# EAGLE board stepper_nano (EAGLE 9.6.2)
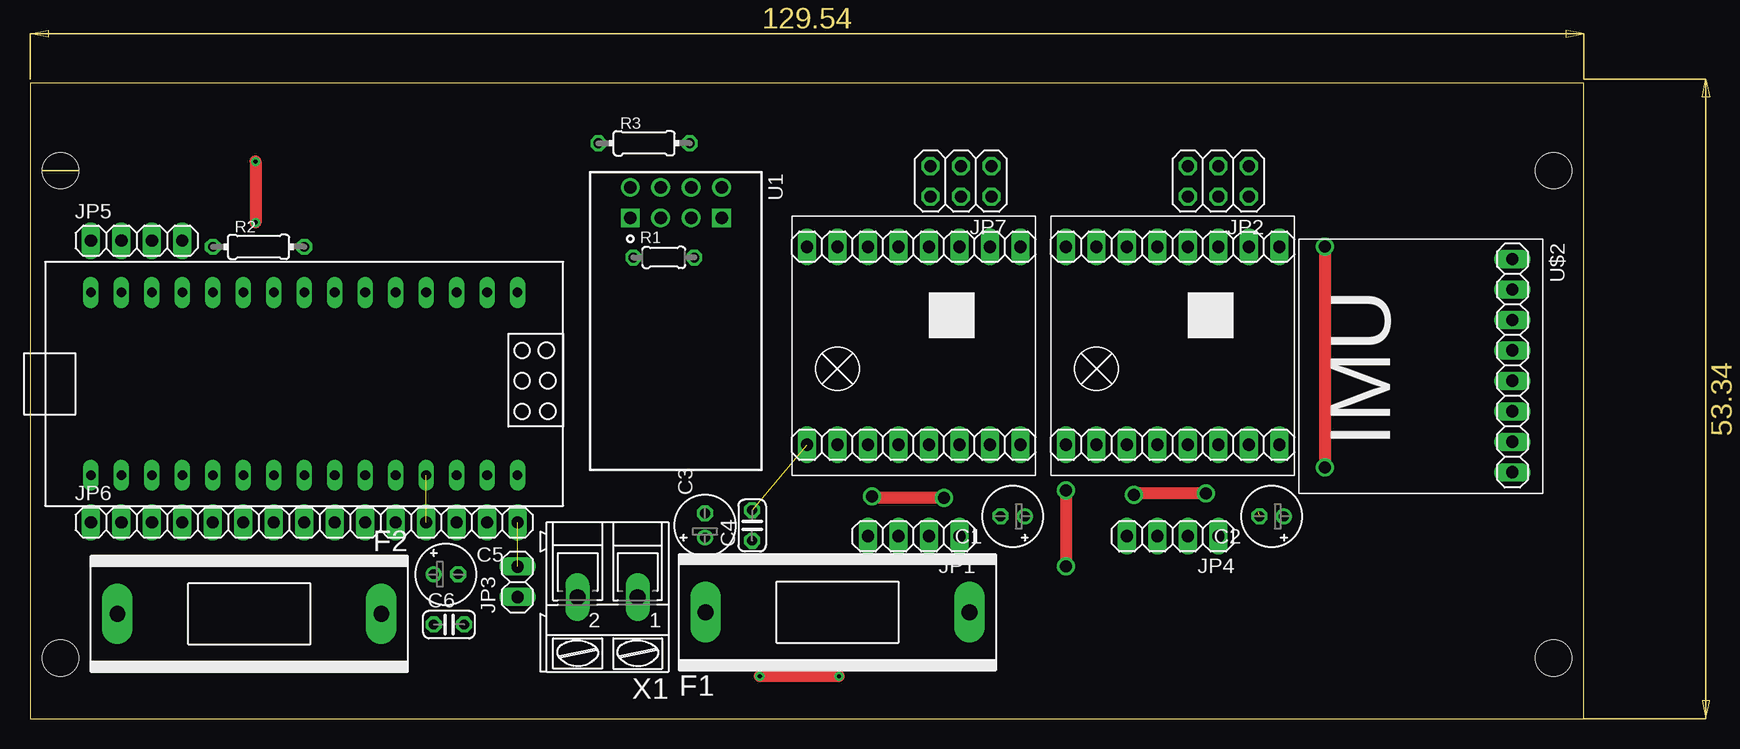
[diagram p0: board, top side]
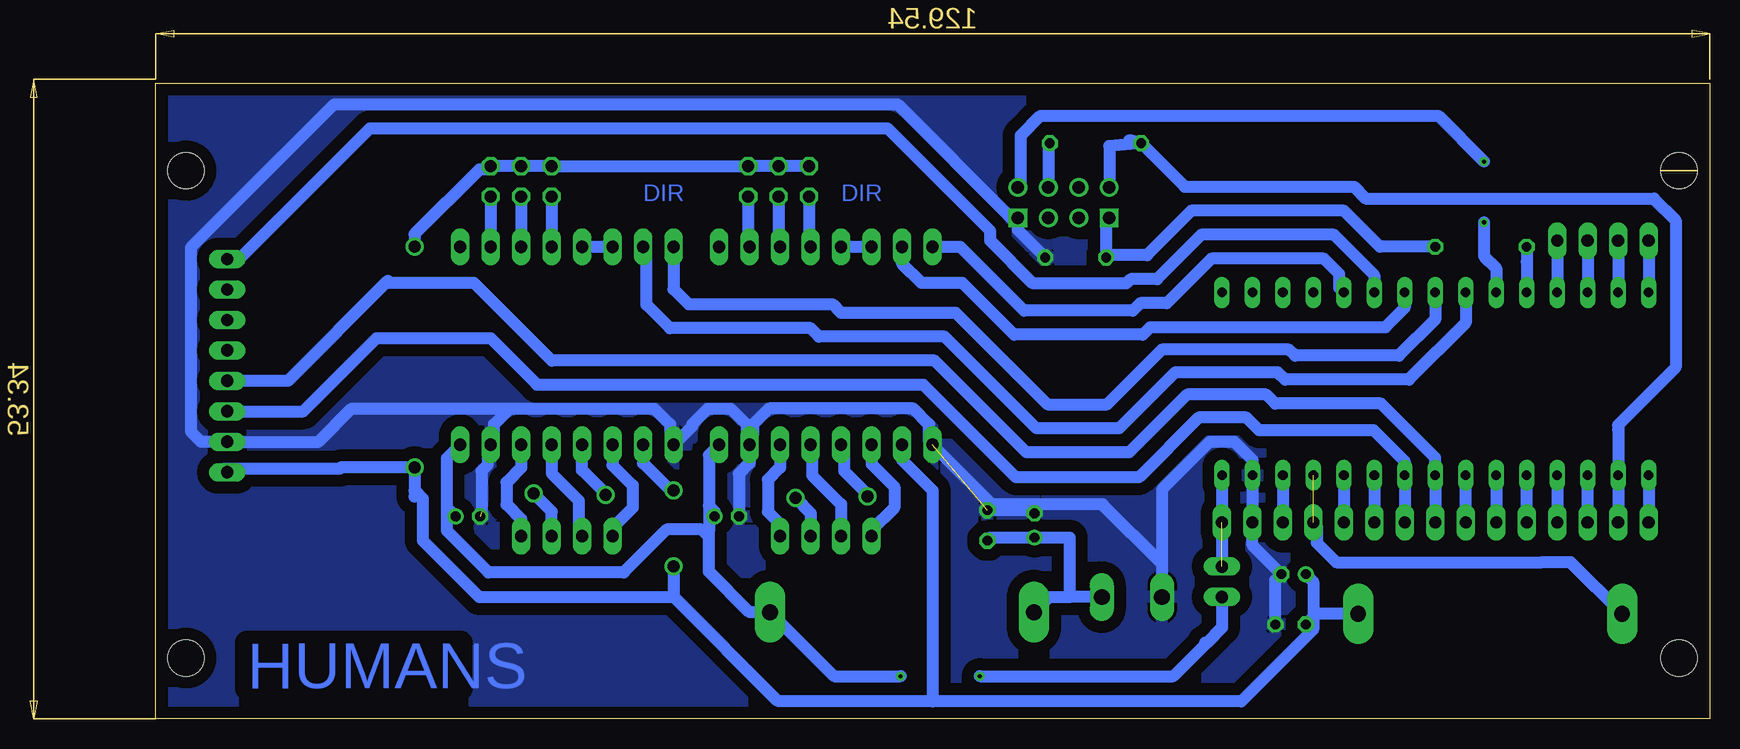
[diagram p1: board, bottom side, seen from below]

Size 140 x 57.45 mm. Coordinates in mm from the lower left corner, seen from the top.
Outline: 0,0 129.52,0 129.52,53.01 0,53.01 0,0
Copper layers (1*16): Top 0.035mm / dielectric 1.5mm / Bottom 0.035mm
Design rules "default *": minimum track width 6mil, minimum drill 0.35mm, track to track 1mm, track to pad 1mm, pad to pad 1mm, via to via 6mil, smd to smd 6mil, copper to edge 40mil, drill to drill 6mil, minimum pad ring 10mil, minimum via ring 8mil, stop-mask expansion 4mil, vias tented up to drill 0mil, thermal gap 10mil
Holes 3 mm at 2.54,45.72 2.54,5.08 127,5.08 127,45.72

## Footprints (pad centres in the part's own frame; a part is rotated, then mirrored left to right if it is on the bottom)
E2-5 = drill 0.813 pad 1.27: + -1.016,0 | drill 0.813 pad 1.27 octagon: - 1.016,0
C025-024X044 = drill 0.813 octagon: 1 -1.27,0; 2 1.27,0
SH22 = drill 1.321 pad 2.54 long: 1 -10.998,0; 2 10.998,0
1X04 = drill 1.016 long: 1 -3.81,0; 2 -1.27,0; 3 1.27,0; 4 3.81,0
2X03 = drill 1.016 octagon: 1 -2.54,-1.27; 2 -2.54,1.27; 3 0,-1.27; 4 0,1.27; 5 2.54,-1.27; 6 2.54,1.27
1X02 = drill 1.016 long: 1 -1.27,0; 2 1.27,0
1X15 = drill 1.016 long: 1 -17.78,0; 2 -15.24,0; 3 -12.7,0; 4 -10.16,0; 5 -7.62,0; 6 -5.08,0; 7 -2.54,0; 8 0,0; 9 2.54,0; 10 5.08,0; 11 7.62,0; 12 10.16,0; 13 12.7,0; 14 15.24,0; 15 17.78,0
0204/5 = drill 0.813 octagon: 1 -2.54,0; 2 2.54,0
0204/7 = drill 0.813 octagon: 1 -3.81,0; 2 3.81,0
XCVR_ESP8266-01/ESP-01 = drill 1.05 square: 1 0,-3.81; 4 0,3.81 | drill 1.05: 2 0,-1.27; 3 0,1.27; 5 -2.54,3.81; 6 -2.54,1.27; 7 -2.54,-1.27; 8 -2.54,-3.81
NANO = drill 0.8 long: 3.3V -10.16,24.13; 5V -10.16,-1.27; A0 -10.16,19.05; A1 -10.16,16.51; A2 -10.16,13.97; A3 -10.16,11.43; A4 -10.16,8.89; A5 -10.16,6.35; A6 -10.16,3.81; A7 -10.16,1.27; AREF -10.16,21.59; D2 5.08,1.27; D3 5.08,3.81; D4 5.08,6.35; D5 5.08,8.89; D6 5.08,11.43; D7 5.08,13.97; D8 5.08,16.51; D9 5.08,19.05; D10 5.08,21.59; D11 5.08,24.13; D12 5.08,26.67; D13 -10.16,26.67; GND -10.16,-6.35; GND1 5.08,-1.27; RAW -10.16,-8.89; RST -10.16,-3.81; RST1 5.08,-3.81; RX1 5.08,-6.35; TX0 5.08,-8.89
IMU_GY521 = drill 1.016 long: ADO -6.35,0; GND 6.35,0; INT -8.89,0; SCL 3.81,0; SDA 1.27,0; VCC 8.89,0; XCL -3.81,0; XDA -1.27,0
A4988-DRIVER = drill 1.016 long: 1 -7.62,8.89; 2 -7.62,6.35; 3 -7.62,3.81; 4 -7.62,1.27; 5 -7.62,-1.27; 6 -7.62,-3.81; 7 -7.62,-6.35; 8 -7.62,-8.89; 9 8.89,8.89; 10 8.89,6.35; 11 8.89,3.81; 12 8.89,1.27; 13 8.89,-1.27; 14 8.89,-3.81; 15 8.89,-6.35; 16 8.89,-8.89
AK300/2 = drill 1.321 long: 1 -2.515,0; 2 2.489,0

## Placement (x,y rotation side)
C1  [E2-5]  81.92,16.89 180 top
C2  [E2-5]  103.5,16.89 180 top
C3  [E2-5]  56.26,16.13 90 top
C4  [C025-024X044]  60.2,16.13 90 top
C5  [E2-5]  34.67,12.07 0 top
C6  [C025-024X044]  34.92,7.87 0 top
F1  1A  [SH22]  67.31,8.89 0 top
F2  300mA  [SH22]  18.29,8.76 180 top
JP1  [1X04]  73.66,15.24 180 top
JP2  [2X03]  99.06,44.83 180 top
JP3  [1X02]  40.64,11.43 90 top
JP4  [1X04]  95.25,15.24 180 top
JP5  [1X04]  8.89,39.88 0 top
JP6  [1X15]  22.86,16.38 0 top
JP7  [2X03]  77.6,44.83 180 top
R1  [0204/5]  52.83,38.48 0 top
R2  [0204/7]  19.05,39.37 0 top
R3  [0204/7]  51.18,48.01 0 top
U1  ESP8266-01/ESP-01  [XCVR_ESP8266-01/ESP-01]  53.85,41.78 270 top
U$1  ARDUINO_NANO  [NANO]  31.75,30.48 90 top
U$2  IMU-MPU  [IMU_GY521]  123.57,29.46 270 top
U$3  [A4988-DRIVER]  73.66,31.75 270 top
U$4  [A4988-DRIVER]  95.25,31.75 270 top
X1  [AK300/2]  48.13,10.16 180 top

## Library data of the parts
C1-C6 = rcl; SPICEPREFIX: C
F1 F2 = fuse; OC_FARNELL: unknown; OC_NEWARK: unknown
JP1-JP7 = pinhead
R1-R3 = rcl; SPICEPREFIX: R
U1 = mohamed-eagle; AVAILABILITY: Not in stock; DESCRIPTION: MakerFocus 4pcs ESP8266 ESP-01 Serial Wireless WiFi Transceiver Receiver Module 1MB SPI Flash DC3.0-3.6V Internet of Things WiFi Module Board Compatible with Ar duino; MF: AI-Thinker; MP: ESP8266-01/ESP-01; PACKAGE: Non-Standard AI-Thinker; PRICE: None
U$1-U$4 = mohamed-eagle
X1 = con-ptr500; OC_FARNELL: unknown; OC_NEWARK: unknown

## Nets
3.3V: JP6.2 R3.1 U1.8 U$1.3.3V
5V: C5.+ C6.1 F2.1 JP2.1 JP2.3 JP2.5 JP7.1 JP7.3 JP7.5 U$2.VCC U$3.15 U$4.15
BAT+12: C1.+ C2.+ F1.2 JP3.1 U$3.9 U$4.9
D7: U1.5 U$1.D7
D8: R2.1 U$1.D8
DIR: U$1.D2 U$3.8
DIR1: U$1.D5 U$4.8
FUSE-5V: F2.2 JP6.12 U$1.5V
GND: C1.- C2.- C3.- C4.2 C5.- C6.2 JP6.14 R1.2 U1.4 U$1.GND U$2.GND U$3.10 U$3.16 U$4.10 U$4.16 X1.2
IMU-INT: U$1.D3 U$2.INT
N$1: JP1.1 U$3.11
N$2: JP1.4 U$3.14
N$3: JP1.2 U$3.13
N$4: JP1.3 U$3.12
N$5: JP4.1 U$4.11
N$6: JP4.4 U$4.14
N$7: JP4.2 U$4.13
N$8: JP4.3 U$4.12
N$9: JP7.2 U$3.2
N$10: JP7.4 U$3.3
N$11: JP7.6 U$3.4
N$12: U$3.5 U$3.6
N$13: JP2.2 U$4.2
N$14: JP2.4 U$4.3
N$15: JP2.6 U$4.4
N$16: U$4.5 U$4.6
N$17: R3.2 U1.6
N$18: JP3.2 JP6.15 U$1.RAW
N$19: JP5.4 U$1.D9
N$20: JP5.3 U$1.D10
N$21: R1.1 R2.2 U1.1
N$22: JP5.2 U$1.D11
N$23: JP5.1 U$1.D12
N$24: JP6.1 U$1.D13
N$25: JP6.3 U$1.AREF
N$26: JP6.4 U$1.A0
N$27: JP6.5 U$1.A1
N$28: JP6.6 U$1.A2
N$29: JP6.7 U$1.A3
N$30: JP6.10 U$1.A6
N$31: JP6.11 U$1.A7
N$32: JP6.13 U$1.RST
N$34: C3.+ C4.1 F1.1 X1.1
SCL: JP6.9 U$1.A5 U$2.SCL
SDA: JP6.8 U$1.A4 U$2.SDA
STEP: U$1.D4 U$3.7
STEP1: U$1.D6 U$4.7

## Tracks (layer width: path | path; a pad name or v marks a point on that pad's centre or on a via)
3.3V
  Bottom 1: R3.1 50.04,47.76 U1.8 | R3.1 48.39,48.26 | 7.62,24.13 U$1.3.3V | U$1.3.3V JP6.2 | R3.1 43.73,44.37 29.64,44.37 28.68,43.4 4.64,43.4 2.82,41.58 2.82,29.31 7.62,24.51 U$1.3.3V
5V  (via drill 1)
  Top 1: v86.36,19.05 v86.36,12.7 | v107.95,39.37 v107.95,20.99
  Bottom 1: 33.02,7.62 33.02,11.43 C5.+ | 33.02,7.62 33.02,7.46 39.04,1.45 64.77,1.45 64.77,1.52 | JP7.5 JP7.3 JP7.1 JP2.5 JP2.3 JP2.1 101.88,45.82 102.54,45.82 107.95,40.41 v107.95,39.37 | U$4.15 88.9,21.34 86.61,19.05 v86.36,19.05 | v86.36,12.7 86.36,10.16 | U$2.VCC 123.85,20.85 114.16,20.85 114.02,20.99 v107.95,20.99 107.95,19.05 | 107.95,19.05 107.95,18.54 | 33.02,7.62 33.4,7.62 C6.1 32.77,8.76 F2.1 | U$3.15 67.31,21.59 64.77,19.05 64.77,1.52 | 107.95,19.05 107.26,18.36 107.26,14.87 102.55,10.16 86.36,10.16 | 86.36,10.16 77.72,1.52 64.77,1.52
BAT+12  (via drill 0.35)
  Top 1: v67.44,3.56 v60.83,3.56
  Bottom 1: 41.91,6.35 42.04,6.35 | 103.86,23.14 U$4.9 105.26,21.74 105.26,17.63 | U$3.9 83.42,22 83.42,17.78 | 105.26,17.63 105.26,15.7 101.78,12.22 90.5,12.22 86.92,15.8 84.02,15.8 83.64,15.42 83.42,15.65 | C2.+ 105.26,17.63 | 83.42,17.78 83.42,15.65 | C1.+ 82.93,17.3 83.42,17.78 | 83.42,15.65 83.42,12.3 80.01,8.89 F1.2 72.97,3.56 v67.44,3.56 | v60.83,3.56 44.7,3.56 41.91,6.35 | JP3.1 40.64,7.62 41.91,6.35
D7  (via drill 0.35)
  Top 1: v18.8,46.48 v18.8,41.4
  Bottom 1: U$1.D7 17.78,37.59 18.8,38.6 v18.8,41.4 | U1.5 57.41,44.57 57.41,48.65 55.76,50.29 22.61,50.29 v18.8,46.48
D8
  Bottom 1: R2.1 15.24,38.1 U$1.D8
DIR
  Bottom 1: U$1.D2 30.87,35.95 30.87,37.11 32.13,38.37 41.53,38.37 45.23,34.67 47.44,34.67 48.08,34.04 57.14,34.04 62.47,39.37 U$3.8
DIR1
  Bottom 1: U$1.D5 22.86,33.3 25.88,30.29 34.54,30.29 35.05,30.8 45.66,30.8 50.23,26.23 55.18,26.23 62.84,33.88 72.43,33.88 73.12,34.58 85.09,34.58 86.36,35.84 U$4.8
FUSE-5V  (1 unrouted)
  Bottom 1: JP6.12 32.74,16.11 32.74,14.68 31.11,13.06 13.97,13.06 11.58,13.06 F2.2
GND  (2 unrouted)
  Bottom 1: 100,25.88 101.32,24.56 101.32,23.14 U$4.10 101.86,22.6 101.86,21.18 102.36,20.68 102.36,17.27 | 100,25.88 87.96,25.88 86.64,24.56 86.64,23.14 U$4.16 84.81,24.41 84.81,24.56 83.49,25.88 81.61,25.88 80.27,24.54 80.27,23.12 | 80.27,23.12 U$3.10 80.01,21.34 80.9,20.45 C1.- | 100,25.88 113.18,25.88 115.95,23.11 U$2.GND 125.73,23.11 126.59,23.98 126.59,39.29 114.63,51.25 67.7,51.25 58.23,41.78 U1.4 57.66,40.77 R1.2 | 80.27,23.12 79.73,23.66 79.73,24.56 78.41,25.88 66.37,25.88 65.05,24.56 65.05,23.14 U$3.16 59.82,17.91 50.6,17.91 45.64,12.95 X1.2 | X1.2 45.64,19.13 41.64,23.13 39.64,23.13 38.1,21.59 U$1.GND JP6.14 38.1,14.48 C5.- 36.2,11.56 C6.2 | X1.2 45.64,10.94 | C3.- 56.52,17.4 C4.2
  pour Bottom: 0,53.34 129.54,53.34 129.54,0 0,0
IMU-INT
  Bottom 1: 123.29,38.08 U$2.INT 122.56,38.35 111.66,49.25 68.53,49.25 59.94,40.66 59.95,40.65 59.95,39.87 56.39,36.32 48.62,36.32 48.27,36.67 46.06,36.67 42.36,40.37 31.3,40.37 27.94,37.01 U$1.D3
N$1
  Bottom 1: U$3.11 77.47,20.95 78.49,19.94 78.49,17.27 77.47,16.26 JP1.1
N$2
  Bottom 1: JP1.4 69.85,15.7 67.94,17.61 67.94,19.35 69.85,21.25 U$3.14
N$3  (via drill 1)
  Top 1: v76.2,18.41 70.32,18.41 v70.19,18.54
  Bottom 1: v76.2,18.41 74.93,17.15 JP1.2 | v70.19,18.54 70.19,18.74 72.11,20.65 72.11,22.58 U$3.13
N$4
  Bottom 1: U$3.12 74.8,22.73 74.8,20.32 72.39,17.91 JP1.3
N$5
  Bottom 1: U$4.11 99.06,20.96 100.29,19.74 100.29,17.87 99.06,16.65 JP4.1
N$6
  Bottom 1: JP4.4 91.44,15.93 89.76,17.61 89.76,19.47 91.44,21.16 U$4.14
N$7  (via drill 1)
  Top 1: v98.04,18.8 92.14,18.8 v92.01,18.67
  Bottom 1: JP4.2 96.52,17.29 v98.04,18.8 | v92.01,18.67 92.01,18.79 93.98,20.76 U$4.13
N$8
  Bottom 1: JP4.3 94.26,15.52 94.26,18.21 96.52,20.47 U$4.12
N$9
  Bottom 1: JP7.2 80.14,39.5 U$3.2
N$10
  Bottom 1: JP7.4 77.6,39.5 U$3.3
N$11
  Bottom 1: JP7.6 75.06,39.5 U$3.4
N$12
  Bottom 1: U$3.5 U$3.6
N$13
  Bottom 1: JP2.2 U$4.2
N$14
  Bottom 1: JP2.4 U$4.3
N$15
  Bottom 1: JP2.6 U$4.4
N$16
  Bottom 1: U$4.5 U$4.6
N$17
  Bottom 1: R3.2 55.12,47.99 U1.6
N$18  (1 unrouted)
  Bottom 1: U$1.RAW JP3.2
N$19
  Bottom 1: JP5.4 U$1.D9
N$20
  Bottom 1: JP5.3 U$1.D10
N$21
  Bottom 1: U1.1 50.29,41.78 R1.1 50.1,38.67 46.89,38.67 43.19,42.37 30.47,42.37 27.47,39.37 R2.2
N$22
  Bottom 1: JP5.2 U$1.D11
N$23
  Bottom 1: JP5.1 U$1.D12
N$24
  Bottom 1: U$1.D13 JP6.1
N$25
  Bottom 1: JP6.3 U$1.AREF
N$26
  Bottom 1: U$1.A0 JP6.4
N$27
  Bottom 1: JP6.5 U$1.A1
N$28
  Bottom 1: U$1.A2 JP6.6
N$29
  Bottom 1: JP6.7 U$1.A3
N$30
  Bottom 1: U$1.A6 JP6.10
N$31
  Bottom 1: U$1.A7 JP6.11
N$32
  Bottom 1: U$1.RST JP6.13
N$34
  Bottom 1: X1.1 53.34,10.16 | F1.1 55.04,10.16 53.34,10.16 | C4.1 59.94,15.11 C3.+ 53.34,15.11 53.34,10.16
SCL
  Bottom 1: U$2.SCL 117.22,25.65 111.12,31.75 101.6,31.75 97.73,27.88 65.55,27.88 57.81,20.15 47.58,20.15 42.6,25.13 38.6,25.13 37.54,24.07 27.99,24.07 25.41,21.48 U$1.A5 JP6.9
SDA
  Bottom 1: JP6.8 U$1.A4 22.86,21.77 27.38,26.29 36.2,26.29 36.96,27.05 43.56,27.05 48.39,22.23 56.93,22.23 64.59,29.88 96.52,29.88 102.98,36.35 110.01,36.35 110.17,36.51 118.49,28.19 U$2.SDA
STEP
  Bottom 1: 67.18,39.24 U$3.7 67.31,37.95 65.71,36.35 62.28,36.35 57.97,32.04 47.25,32.04 46.61,32.67 27.02,32.67 25.4,34.29 U$1.D4
STEP1
  Bottom 1: U$1.D6 20.32,33.02 25.05,28.29 35.37,28.29 36,28.92 44.52,28.92 49.22,24.23 56.1,24.23 63.76,31.88 74.24,31.88 74.93,32.58 86.65,32.58 88.62,34.55 88.62,39.09 U$4.7

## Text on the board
Bottom: DIR | DIR | HUMANS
